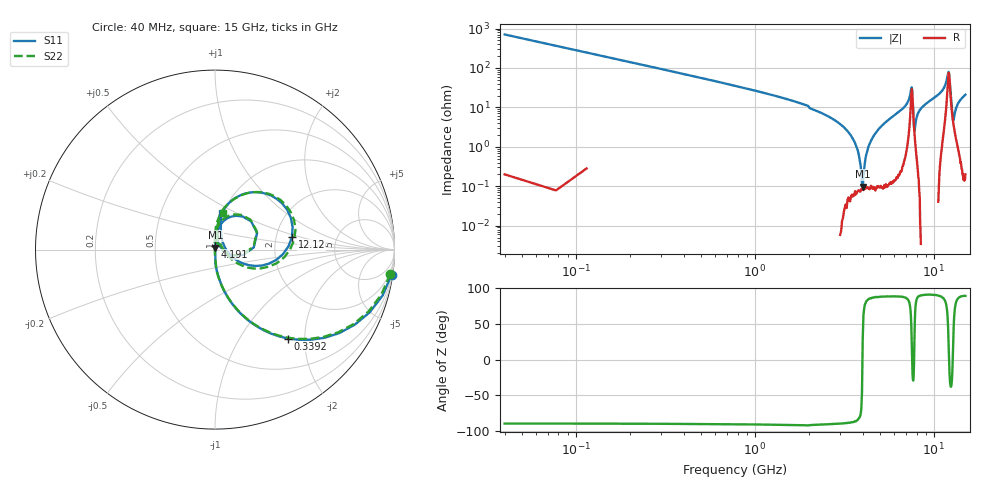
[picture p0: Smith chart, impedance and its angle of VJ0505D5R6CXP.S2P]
! VJ0505D5R6CXP
! MLCC placed on 25 mil thick microstrip substrate in series configuraton.
! DATE 06/29/2018  07:52
! CORRECTED  DATA
# GHz  S  MA  R  50.00
!  FREQ  S11M  S11A  S21M  S21A  S12M  S12A  S22M  S22A
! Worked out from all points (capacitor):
!   401 points, 40 MHz to 15 GHz, reference 50 ohm
!   read as one part in series: C = 5.63 pF near 114.8 MHz
!   lowest |Z| = 98.4 mohm at 4.004 GHz (marker M1)
!   series resonance near 3.991 GHz, so ESL is about 280 pH
!   S11 on the Smith chart (normalised r, x): 40 MHz: 1, -14; 339.2 MHz: 0.99, -1.66; 4.191 GHz: 1.00, +0.04; 12.12 GHz: 2.45, +0.43; 15 GHz: 0.99, +0.43
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0.04  0.9933 -8.0  0.1402 82.0  0.1407 81.8  0.9857 -8.0
0.1896  0.8342 -33.9  0.5579 56.3  0.5582 56.3  0.8272 -33.8
0.3392  0.6423 -50.5  0.7722 39.9  0.7729 39.9  0.6367 -50.4
0.9002  0.2873 -74.2  0.9629 16.9  0.9633 16.9  0.2855 -74.2
2.5458  0.05284 -87.8  0.9986 3.9  0.9991 3.9  0.0526 -88.2
3.2938  0.0154 -85.0  0.9985 2.0  0.999 2.0  0.01538 -92.6
3.4808  0.007825 -80.3  0.9985 1.6  0.9991 1.6  0.007372 -96.4
3.6678  0.001357 -11.9  0.9986 1.2  0.9991 1.2  0.0011 172.5
4.0044  0.01178 80.9  0.9983 0.6  0.9988 0.6  0.01231 96.9
4.1914  0.01774 82.7  0.998 0.3  0.9987 0.3  0.01832 95.7
5.0516  0.04561 85.3  0.9972 -1.1  0.9976 -1.0  0.0453 91.5
7.1086  0.1412 78.0  0.979 -6.4  0.9798 -6.4  0.1426 81.2
7.52  0.2525 21.6  0.7684 -5.0  0.769 -5.0  0.2543 23.6
7.7818  0.03411 43.5  0.976 0.3  0.9767 0.3  0.03135 50.8
8.3428  0.09823 83.2  0.9937 -4.0  0.9944 -4.0  0.1008 88.6
10.0258  0.1837 81.2  0.9839 -9.1  0.9851 -9.0  0.1891 82.4
11.7836  0.396 53.9  0.8132 -21.4  0.8137 -21.4  0.4076 51.8
12.1202  0.4348 9.4  0.5676 -4.0  0.568 -4.0  0.444 6.9
12.5316  0.1164 -24.4  0.9028 4.7  0.9032 4.7  0.1085 -30.4
12.7934  0.05541 23.4  0.956 0.0  0.9566 0.0  0.04071 32.7
13.504  0.121 74.9  0.9806 -5.8  0.9815 -5.8  0.1213 83.6
15  0.2092 78.6  0.9752 -11.4  0.9755 -11.4  0.2103 77.7
